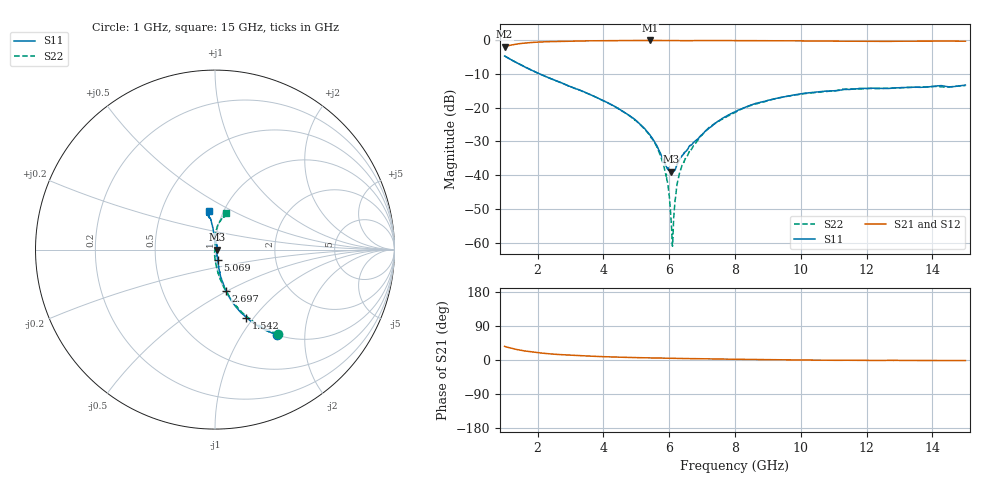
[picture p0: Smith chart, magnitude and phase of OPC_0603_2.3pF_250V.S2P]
! FILE NAME
! DATE 08/15/2012  10:11
! CORRECTED  DATA
# GHz  S  MA  R  50.00
!  FREQ  S11M  S11A  S21M  S21A  S12M  S12A  S22M  S22A
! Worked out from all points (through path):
!   1601 points, 1 GHz to 15 GHz, reference 50 ohm
!   highest |S21| = -0.06 dB at 5.419 GHz (marker M1); lowest = -1.9 dB at 1 GHz (marker M2)
!   group delay of S21, straight-line fit = 4.6 ps
!   lowest |S11| = -38.9 dB at 6.066 GHz (marker M3), VSWR 1.02, Z = 51.1 - j0.00166 ohm
!   |S11| at or under -10 dB: 2.074 GHz to end of sweep
!   |S22| runs from -61.0 to -4.7 dB; largest |S21 - S12| = 0.0082
!   S11 on the Smith chart (normalised r, x): 1 GHz: 1.00, -1.45; 1.542 GHz: 1.00, -0.92; 2.697 GHz: 1.01, -0.49; 5.069 GHz: 1.02, -0.12; 15 GHz: 0.85, +0.38
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1  0.5854 -54.0  0.8039 35.9  0.8037 35.9  0.5852 -53.4
1.5425  0.4177 -65.2  0.9018 24.9  0.9012 24.9  0.4178 -64.2
2.6975  0.237 -74.8  0.9641 14.2  0.9638 14.2  0.2359 -75.2
3.33625  0.1781 -77.3  0.9775 11.2  0.9767 11.2  0.1773 -78.8
4.3775  0.1026 -78.5  0.9889 7.8  0.9885 7.8  0.1022 -85.1
5.06875  0.05988 -76.0  0.9921 6.1  0.9917 6.2  0.05916 -88.9
5.41875  0.03917 -72.5  0.9935 5.4  0.9925 5.4  0.03809 -92.5
5.6725  0.02435 -65.1  0.993 4.9  0.9928 4.9  0.02321 -95.8
5.9175  0.0133 -36.0  0.9922 4.4  0.9911 4.4  0.01032 -93.2
5.97875  0.01189 -22.4  0.9908 4.4  0.9901 4.4  0.006128 -102.3
6.06625  0.01134 -0.1  0.9901 4.2  0.9898 4.2  0.001866 -107.3
6.10125  0.01169 7.1  0.9901 4.2  0.9893 4.2  0.0008877 -179.0
6.13625  0.0115 15.6  0.9898 4.1  0.9895 4.2  0.002306 113.1
6.215  0.01341 34.2  0.9895 4.0  0.9887 4.0  0.00582 92.1
6.3025  0.01647 44.7  0.9884 3.9  0.9878 3.9  0.01017 83.2
6.55625  0.02403 62.5  0.9873 3.8  0.9871 3.7  0.0195 83.9
7.15125  0.04697 85.1  0.9905 3.1  0.99 3.1  0.04769 90.2
8  0.08731 93.8  0.9886 1.9  0.9877 2.0  0.08501 89.3
9.05  0.1303 96.1  0.9837 0.9  0.9828 0.9  0.1296 84.4
10.33625  0.1681 97.9  0.9774 -0.2  0.9765 -0.2  0.1661 78.8
12.6725  0.1932 102.1  0.9622 -0.9  0.9622 -1.0  0.1945 73.8
15  0.2178 99.5  0.9685 -1.5  0.9681 -1.5  0.213 73.9
